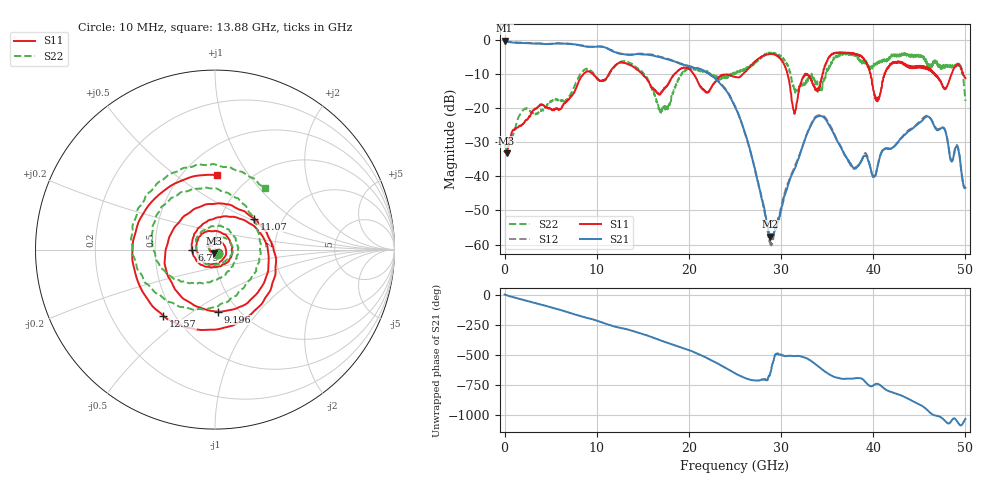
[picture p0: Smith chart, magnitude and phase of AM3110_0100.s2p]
# Hz S DB R 50.0
!freq dBS11 angS11 dBS21 angS21 dBS12 angS12 dBS22 angS22
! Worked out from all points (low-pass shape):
!   1601 points, 10 MHz to 50 GHz, reference 50 ohm
!   highest |S21| = -0.19 dB at 10 MHz (marker M1); lowest = -57.7 dB at 28.79 GHz (marker M2)
!   |S21| within 3 dB of the highest: start of sweep to 11.64 GHz
!   lowest |S11| = -33.2 dB at 228.7 MHz (marker M3), VSWR 1.04, Z = 49.2 - j2.04 ohm
!   |S11| at or under -10 dB: start of sweep to 8.555 GHz; 14.95 GHz to 18.41 GHz (3.455 GHz wide, 20.7 % of centre); 20.52 GHz to 25.87 GHz (5.344 GHz wide, 23 % of centre)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
!   |S22| runs from -32.6 to -3.7 dB; largest |S21 - S12| = 0.024
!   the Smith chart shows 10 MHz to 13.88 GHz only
!   S11 on the Smith chart (normalised r, x): 10 MHz: 1.03, -0.04; 6.79 GHz: 0.77, -0.00; 9.196 GHz: 0.81, -0.64; 11.07 GHz: 1.44, +0.54; 12.57 GHz: 0.44, -0.41; 13.88 GHz: 0.72, +0.72
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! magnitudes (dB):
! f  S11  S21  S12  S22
! 10 MHz  -32.7  -0.2  -0.1  -30.4
! 228.7 MHz  -33.2  -0.3  -0.3  -32.2
! 2.072 GHz  -24.4  -0.9  -0.8  -20.4
! 6.79 GHz  -17.7  -1.1  -1.0  -17.3
! 8.352 GHz  -10.7  -1.7  -1.5  -9.5
! 9.196 GHz  -9.2  -2.0  -2.0  -8.6
! 11.07 GHz  -11.1  -2.3  -2.3  -11.4
! 12.57 GHz  -6.6  -4.0  -3.9  -6.4
! 13.88 GHz  -7.7  -4.3  -4.2  -7.1
! 16.69 GHz  -15.8  -4.9  -4.7  -19.4
! 19.82 GHz  -8.2  -7.5  -7.5  -8.4
! 25 GHz  -10.8  -19.6  -19.4  -9.6
! 28.79 GHz  -4.1  -57.7  -59.0  -3.7
! 30.38 GHz  -7.4  -45.8  -45.0  -5.7
! 31.41 GHz  -20.8  -38.1  -37.7  -14.4
! 33.35 GHz  -12.0  -24.5  -24.2  -9.9
! 37.63 GHz  -3.8  -36.7  -37.1  -4.0
! 40.03 GHz  -14.8  -39.9  -40.4  -7.7
! 41.69 GHz  -7.7  -31.9  -31.8  -5.8
! 45.97 GHz  -8.3  -22.5  -22.3  -8.0
! 49.34 GHz  -7.4  -33.6  -33.4  -7.0
! 50 GHz  -11.2  -43.3  -43.0  -17.9
